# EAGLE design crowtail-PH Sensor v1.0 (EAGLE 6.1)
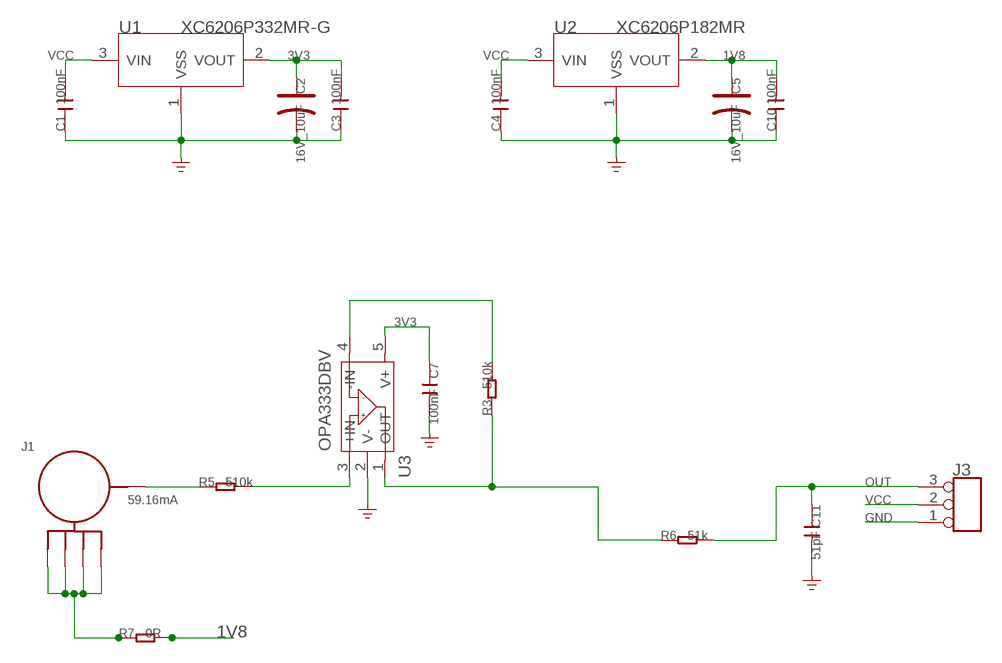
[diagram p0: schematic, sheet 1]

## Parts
C1  100nF  C-0603  [C0603]
C2  16V_10uF  CAP-AVX-A  [AVX-A]
C3  100nF  C-0603  [C0603]
C4  100nF  C-0603  [C0603]
C5  16V_10uF  CAP-AVX-A  [AVX-A]
C7  100nF  C-0603  [C0603]
C10  100nF  C-0603  [C0603]
C11  51pF  C-0603  [C0603]
J1  BNC  [BNC]
J3  TINKER_3P_DIP  [3P_2.0_DIP]
R3  510k  R-0603  [R0603]
R5  510k  R-0603  [R0603]
R6  51k  R-0603  [R0603]
R7  0R  R-0603  [R0603]
U1  XC6206P332MR-G  XC6206MR  [SOT23]
U2  XC6206P182MR  XC6206MR  [SOT23]
U3  OPA333DBV  [SOT23-5]

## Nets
1V8: C5.+ C10.2 R7.2 U2.2(VOUT)
3V3: C2.+ C3.2 C7.1 U1.2(VOUT) U3.5(V+)
GND: C1.1 C2.- C3.1 C4.1 C5.- C7.2 C10.1 C11.2 J3.1 U1.1(VSS) U2.1(VSS) U3.2(V-)
N$1: J1.P$1 R5.1
N$2: R5.2 U3.3(+IN)
N$3: R3.1 R6.1 U3.1(OUT)
N$4: R3.2 U3.4(-IN)
N$6: J1.P$2 J1.P$3 J1.P$4 J1.P$5 R7.1
OUT: C11.1 J3.3 R6.2
VCC: C1.2 C4.2 J3.2 U1.3(VIN) U2.3(VIN)

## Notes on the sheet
- 59.16mA

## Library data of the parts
C1 C3 C4 C7 C10 C11 = Discrete:C*: Ceramic Capacitors
C2 C5 = Discrete:CAP*: Electrolytic Capacitors,Tantalum Capacitors and Super Capacitors
J1 = BNC:BNC
J3 = Connector:TINKER_3P_DIP
R3 R5-R7 = Discrete:R*
U1 U2 = IC:XC6206: LOW ESR Cap.Compatible Positive Voltage Regulators
U3 = IC:OPA333: 1.8V,Micro power CMOS oprational amplifiers Zero-Drift Series http://www.ti.com.cn/cn/lit/ds/symlink/opa333.pdf

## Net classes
0 default: width 0.152 mm, drill 0.305 mm, clearance 0.152 mm

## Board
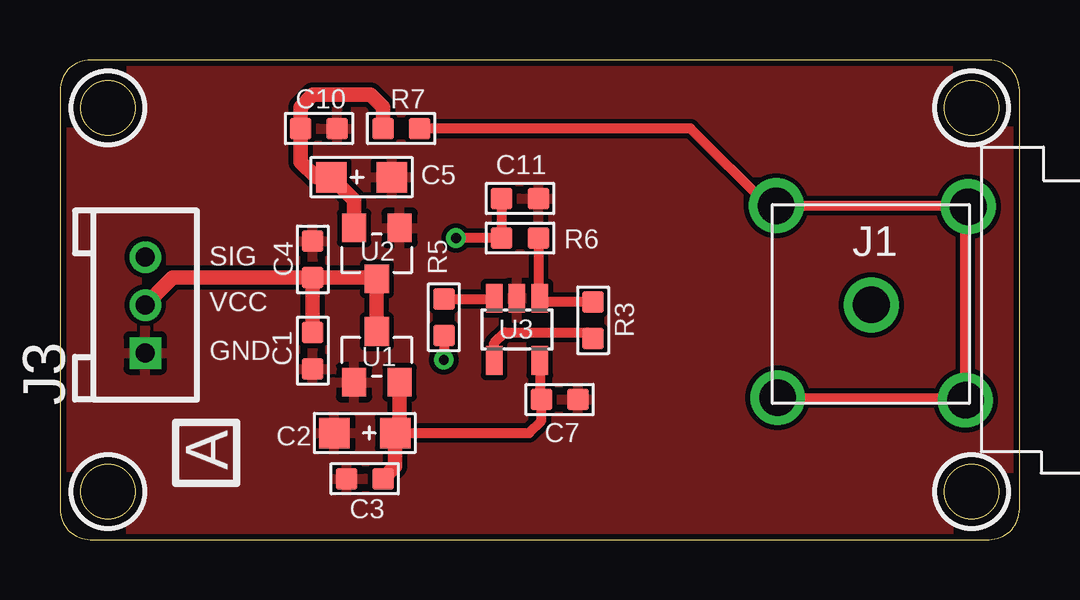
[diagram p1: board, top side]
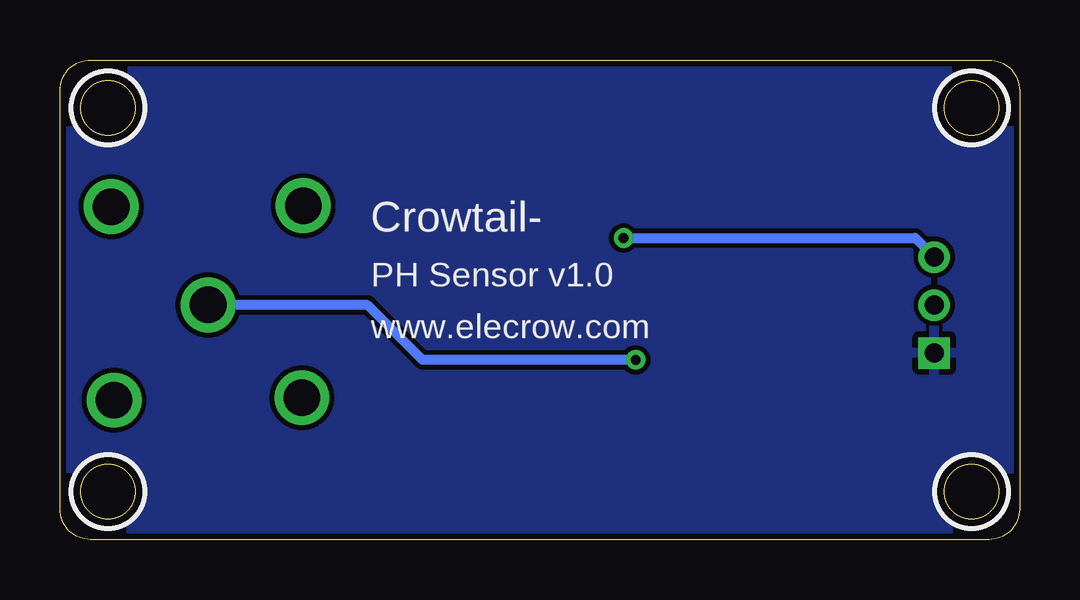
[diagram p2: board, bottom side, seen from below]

Size 40 x 20 mm. Coordinates in mm from the lower left corner, seen from the top.
Outline: 0,18.73 0,1.27 arc90 1.27,0 38.73,0 arc90 40,1.27 40,18.73 arc90 38.73,20 1.27,20 arc90 0,18.73
Outline: circle at 2,18 radius 1.14
Outline: circle at 38,2 radius 1.14
Outline: circle at 2,2 radius 1.14
Outline: circle at 38,18 radius 1.14
Copper layers (1*16): Top 0.035mm / dielectric 1.5mm / Bottom 0.035mm
Design rules: minimum track width 10mil, minimum drill 12mil, track to track 8mil, track to pad 8mil, pad to pad 8mil, via to via 8mil, smd to smd 0mil, copper to edge 10mil, drill to drill 8mil, minimum pad ring 10mil, minimum via ring 8mil, stop-mask expansion 4mil, vias tented up to drill 100mil, thermal gap 10mil
tRestrict: area 0.5,16.5 to 3.5,19.5; area 36.5,0.5 to 39.5,3.5; area 0.5,0.5 to 3.5,3.5; area 36.5,16.5 to 39.5,19.5
bRestrict: area 0.5,16.5 to 3.5,19.5; area 36.5,0.5 to 39.5,3.5; area 0.5,0.5 to 3.5,3.5; area 36.5,16.5 to 39.5,19.5

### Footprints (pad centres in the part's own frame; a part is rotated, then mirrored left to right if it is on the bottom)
C0603 = smd 0.889 x 0.889: 1 -0.762,0; 2 0.762,0
AVX-A = smd 1.27 x 1.27: + -1.27,0; - 1.27,0
BNC = drill 1.524: P$1 -0.976,0.512; P$2 2.948,-3.456; P$3 -4.94,4.65; P$4 3.068,4.61; P$5 -4.88,-3.356
3P_2.0_DIP = drill 0.8 pad 1.27 square: 1 -2,0 | drill 0.8 pad 1.27: 2 0,0; 3 2,0
R0603 = smd 0.889 x 0.889: 1 -0.762,0; 2 0.762,0
SOT23 = smd 1.016 x 1.2: 1 -0.95,-1.06; 2 0.95,-1.06; 3 0,1.06
SOT23-5 = smd 0.69 x 1.2: 1 -0.95,-1.3; 2 0,-1.3; 3 0.95,-1.3; 4 0.95,1.3; 5 -0.95,1.3

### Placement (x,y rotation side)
C1  10.54,7.87 90 top
C2  12.7,4.45 180 top
C3  12.7,2.54 0 top
C4  10.54,11.68 270 top
C5  12.57,15.11 0 top
C7  20.83,5.84 0 top
C10  10.79,17.14 180 top
C11  19.18,14.22 0 top
J1  34.8,9.27 0 top
J3  3.56,9.78 90 top
R3  22.23,9.14 270 top
R5  16,9.27 90 top
R6  19.18,12.57 180 top
R7  14.22,17.14 180 top
U1  13.21,7.62 0 top
U2  13.21,11.94 180 top
U3  19.05,8.76 180 top

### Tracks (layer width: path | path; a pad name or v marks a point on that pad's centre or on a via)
1V8
  Top 0.61: U2.2 12.26,14.16 C5.+ 10.67,15.11 10.03,15.75 C10.2 10.03,18.03 10.54,18.54 12.95,18.54 13.46,18.03 R7.2
3V3
  Top 0.406: C2.+ 19.56,4.45 20.07,4.95 20.07,5.71 19.94,5.84 20,5.9 20,5.91 | U3.5 20,5.91 | 20,5.91 C7.1
  Top 0.61: C3.2 13.97,3.05 C2.+ 14.16,4.63 U1.2
GND
  pour Top: 38.99,-0.25 0.89,-0.25 arc-90 -0.38,1.02 -0.38,18.92 arc-90 0.89,20.19 38.99,20.19 arc-90 40.26,18.92 40.26,1.02 arc-90
  pour Bottom: 40.26,18.92 40.26,1.02 arc-90 38.99,-0.25 1.02,-0.25 arc-90 -0.25,1.02 -0.25,18.92 arc-90 1.02,20.19 38.99,20.19 arc-90
N$1  (via drill 0.41)
  Top 0.406: R5.1 v16,7.49
  Bottom 0.406: v16,7.49 24.89,7.49 27.18,9.78 J1.P$1
N$2
  Top 0.406: R5.2 18.07,10.03 U3.3
N$3
  Top 0.406: R6.1 19.94,10.12 U3.1 20.16,9.91 R3.1
N$4
  Top 0.406: U3.4 18.1,8.19 18.54,8.64 21.97,8.64 R3.2
N$6
  Top 0.406: R7.1 26.29,17.14 29.51,13.92 J1.P$3 37.83,13.92 J1.P$4 37.75,13.76 J1.P$2 37.65,5.92 J1.P$5
OUT  (via drill 0.41)
  Top 0.406: C11.1 R6.2 v16.51,12.57
  Bottom 0.406: v16.51,12.57 4.35,12.57 J3.3
VCC
  Top 0.61: C4.2 4.7,10.92 J3.2 | C1.2 C4.2 | C4.2 13.16,10.92 U2.3 U1.3

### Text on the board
tPlace: A
bPlace: Crowtail- | PH Sensor v1.0 | www.elecrow.com
tNames: J1 | SIG | VCC | GND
